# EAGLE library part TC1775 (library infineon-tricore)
TC1775 (AUDO1) 32-bit microcontroller for high demanding automotive and industrial applications (e.g. engine management, starter generator, 3-phase motor control or robotics) Source: http://www.infineon.com ..
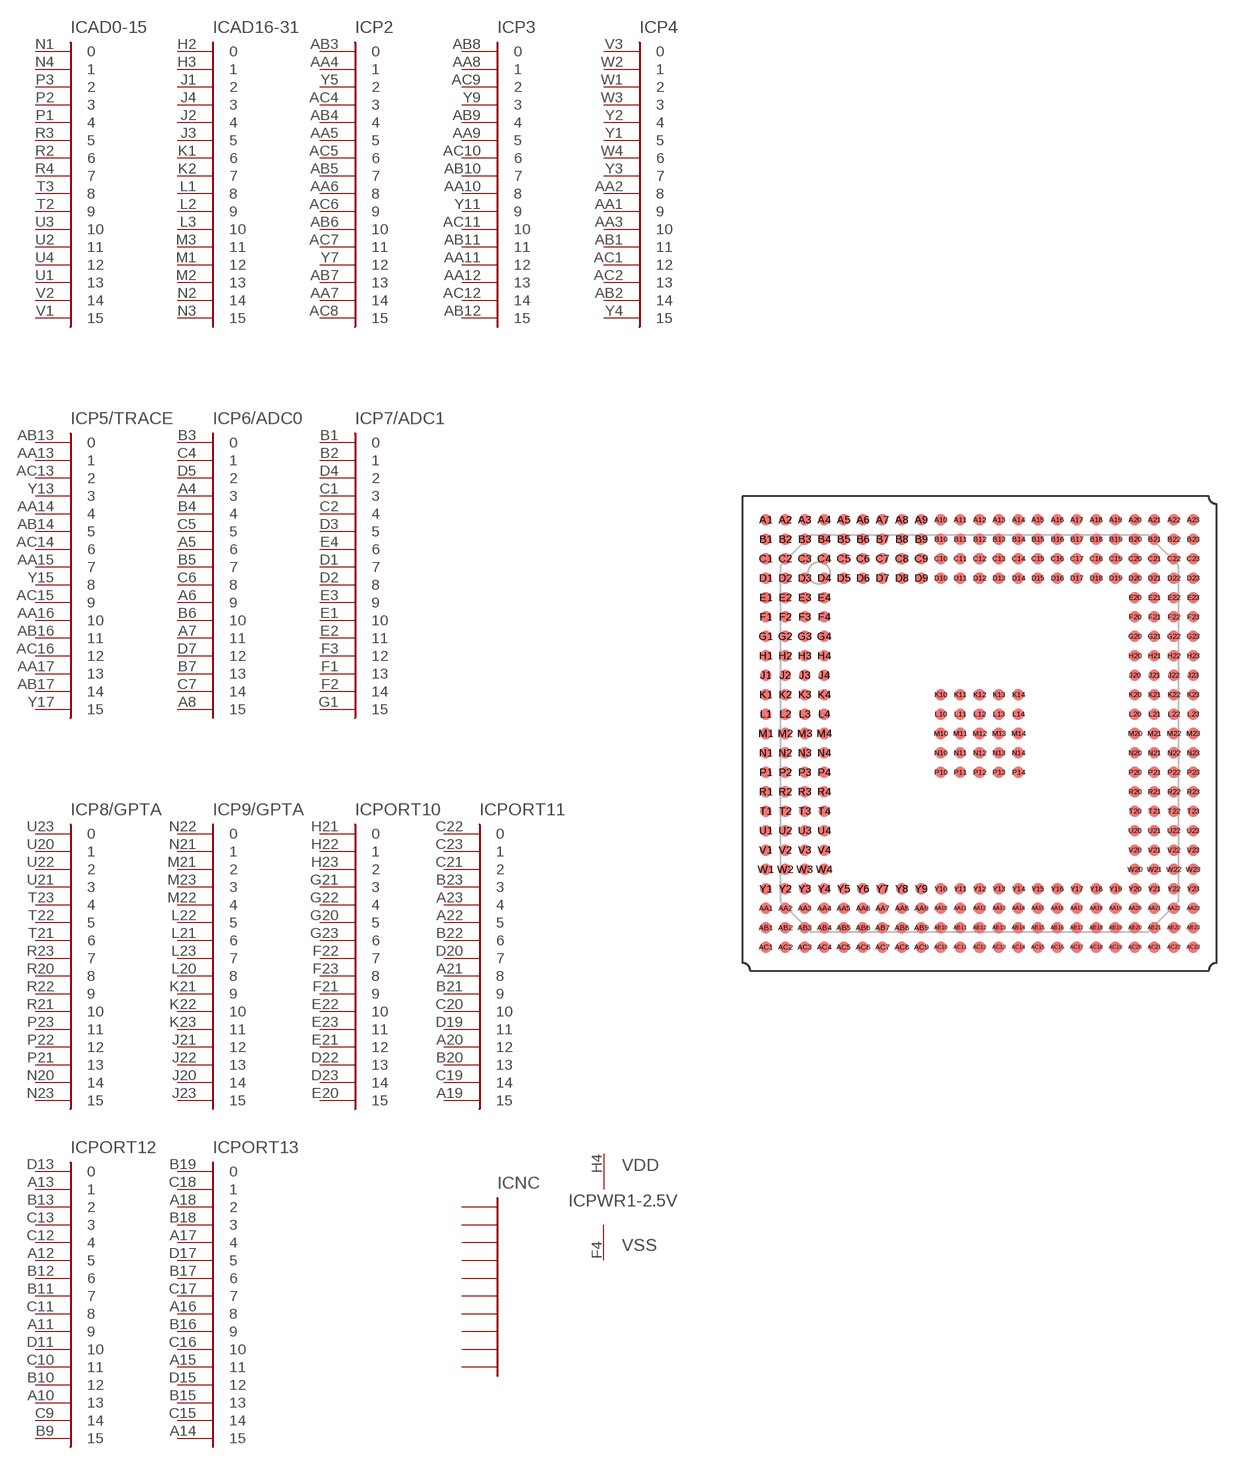
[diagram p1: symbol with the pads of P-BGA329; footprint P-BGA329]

Designator prefix IC; gates PORT12=PORT16 PORT13=PORT16 P8/GPTA=PORT16 P9/GPTA=PORT16 PORT10=PORT16 PORT11=PORT16 P5/TRACE=PORT16 P6/ADC0=PORT16 P7/ADC1=PORT16 AD0-15=PORT16 AD16-31=PORT16 P2=PORT16 P3=PORT16 P4=PORT16 NC=NC10 PWR1-2.5V=VSS_VDD PWR2-2.5V=VSS_VDD PWR3-2.5V=VSS_VDD PWR4-2.5V=VSS_VDD PWR5-2.5V=VSS_VDD PWR6-3.3V=VSS_VDD PWR7-3.3V=VSS_VDD PWR8-3.3V=VSS_VDD PWR9-3.3V=VSS_VDD PWR10-3.3V=VSS_VDD PWR11-3.3V=VSS_VDD PWR12-2.5V=VSS_VDD PWR13-2.5V=VSS_VDD PWR14-2.5V=VSS_VDD PWR15-2.5V=VSS_VDD P-SB-2.5V=VSS_VDD P-SRAM1-2.5V=VSS_VDD P-SRAM2-2.5V=VSS_VDD PWR16-2.5V=VSS_VDD PWR17-2.5V=VSS_VDD PWR18-2.5V=VSS_VDD PWR19-2.5V=VSS_VDD PWR20-2.5V=VSS_VDD PWR21-2.5V=VSS_VDD P-SC-5V=VSS_VDD P-DM-5V=VSS_VDD JTAG=JTAG-OCSD A=TC1775 PWR22=VSS PWR23=VSS PWR24=VSS PWR25=VSS PWR26=VSS

## TC1775 (OC_FARNELL: unknown; OC_NEWARK: unknown)  [P-BGA329]
A1  P-SC-5V:VDD  pwr
A2  P-SC-5V:VSS  pwr
A3  P-SRAM2-2.5V:VSS  pwr
A4  P6/ADC0:3  in
A5  P6/ADC0:6  in
A6  P6/ADC0:9  in
A7  P6/ADC0:11  in
A8  P6/ADC0:15  in
A9  A:VSSA  pwr
A10  PORT12:13  in
A11  PORT12:9  in
A12  PORT12:5  in
A13  PORT12:1  in
A14  PORT13:15  in
A15  PORT13:11  in
A16  PORT13:8  in
A17  PORT13:4  in
A18  PORT13:2  in
A19  PORT11:15  in
A20  PORT11:12  in
A21  PORT11:8  in
A22  PORT11:5  in
A23  PORT11:4  in
AA1  P4:9  in
AA2  P4:8  in
AA3  P4:10  in
AA4  P2:1  in
AA5  P2:5  in
AA6  P2:8  in
AA7  P2:14  in
AA8  P3:1  in
AA9  P3:5  in
AA10  P3:8  in
AA11  P3:12  in
AA12  P3:13  in
AA13  P5/TRACE:1  in
AA14  P5/TRACE:4  in
AA15  P5/TRACE:7  in
AA16  P5/TRACE:10  in
AA17  P5/TRACE:13  in
AA18  JTAG:TDO  out
AA19  JTAG:!TRST  in
AA20  A:XTAL4
AA21  A:VSS  pwr
AA22  A:VDD  pwr
AA23  A:VSS  pwr
AB1  P4:11  in
AB2  P4:14  in
AB3  P2:0  in
AB4  P2:4  in
AB5  P2:7  in
AB6  P2:10  in
AB7  P2:13  in
AB8  P3:0  in
AB9  P3:4  in
AB10  P3:7  in
AB11  P3:11  in
AB12  P3:15  in
AB13  P5/TRACE:0  in
AB14  P5/TRACE:5  in
AB15  NC:NC  nc
AB16  P5/TRACE:11  in
AB17  P5/TRACE:14  in
AB18  P-SRAM2-2.5V:VDD  pwr
AB19  JTAG:TCK  in
AB20  JTAG:TMS  in
AB21  A:XTAL3
AB22  NC:NC  nc
AB23  A:TESTMODE
AC1  P4:12  in
AC2  P4:13  in
AC3  NC:NC  nc
AC4  P2:3  in
AC5  P2:6  in
AC6  P2:9  in
AC7  P2:11  in
AC8  P2:15  in
AC9  P3:2  in
AC10  P3:6  in
AC11  P3:10  in
AC12  P3:14  in
AC13  P5/TRACE:2  in
AC14  P5/TRACE:6  in
AC15  P5/TRACE:9  in
AC16  P5/TRACE:12  in
AC17  P-SRAM1-2.5V:VDD  pwr
AC18  JTAG:!BRKOUT  out
AC19  JTAG:TDI  in
AC20  JTAG:!BRKIN  in
AC21  A:VDD  pwr
AC22  A:XTAL2
AC23  A:XTAL1
B1  P7/ADC1:0  in
B2  P7/ADC1:1  in
B3  P6/ADC0:0  in
B4  P6/ADC0:4  in
B5  P6/ADC0:7  in
B6  P6/ADC0:10  in
B7  P6/ADC0:13  in
B8  A:VAGND  pwr
B9  PORT12:15  in
B10  PORT12:12  in
B11  PORT12:7  in
B12  PORT12:6  in
B13  PORT12:2  in
B14  P-SB-2.5V:VDD  pwr
B15  PORT13:13  in
B16  PORT13:9  in
B17  PORT13:6  in
B18  PORT13:3  in
B19  PORT13:0  in
B20  PORT11:13  in
B21  PORT11:9  in
B22  PORT11:6  in
B23  PORT11:3  in
C1  P7/ADC1:3  in
C2  P7/ADC1:4  in
C3  P-DM-5V:VDD  pwr
C4  P6/ADC0:1  in
C5  P6/ADC0:5  in
C6  P6/ADC0:8  in
C7  P6/ADC0:14  in
C8  A:VAREF  pwr
C9  PORT12:14  in
C10  PORT12:11  in
C11  PORT12:8  in
C12  PORT12:4  in
C13  PORT12:3  in
C14  NC:NC  nc
C15  PORT13:14  in
C16  PORT13:10  in
C17  PORT13:7  in
C18  PORT13:1  in
C19  PORT11:14  in
C20  PORT11:10  in
C21  PORT11:2  in
C22  PORT11:0  in
C23  PORT11:1  in
D1  P7/ADC1:7  in
D2  P7/ADC1:8  in
D3  P7/ADC1:5  in
D4  P7/ADC1:2  in
D5  P6/ADC0:2  in
D6  PWR15-2.5V:VDD  pwr
D7  P6/ADC0:12  in
D8  PWR6-3.3V:VDD  pwr
D9  A:VDDA  pwr
D10  NC:NC  nc
D11  PORT12:10  in
D12  PWR7-3.3V:VDD  pwr
D13  PORT12:0  in
D14  PWR16-2.5V:VDD  pwr
D15  PORT13:12  in
D16  PWR8-3.3V:VDD  pwr
D17  PORT13:5  in
D18  PWR4-2.5V:VSS  pwr
D19  PORT11:11  in
D20  PORT11:7  in
D21  NC:NC  nc
D22  PORT10:13  in
D23  PORT10:14  in
E1  P7/ADC1:10  in
E2  P7/ADC1:11  in
E3  P7/ADC1:9  in
E4  P7/ADC1:6  in
E20  PORT10:15  in
E21  PORT10:12  in
E22  PORT10:10  in
E23  PORT10:11  in
F1  P7/ADC1:13  in
F2  P7/ADC1:14  in
F3  P7/ADC1:12  in
F4  PWR1-2.5V:VSS  pwr
F20  PWR19-2.5V:VDD  pwr
F21  PORT10:9  in
F22  PORT10:7  in
F23  PORT10:8  in
G1  P7/ADC1:15  in
G2  A:VAREF  pwr
G3  A:VSSA  pwr
G4  A:VAGND  pwr
G20  PORT10:5  in
G21  PORT10:3  in
G22  PORT10:4  in
G23  PORT10:6  in
H1  A:VDDA  pwr
H2  AD16-31:0  in
H3  AD16-31:1  in
H4  PWR1-2.5V:VDD  pwr
H20  PWR9-3.3V:VDD  pwr
H21  PORT10:0  in
H22  PORT10:1  in
H23  PORT10:2  in
J1  AD16-31:2  in
J2  AD16-31:4  in
J3  AD16-31:5  in
J4  AD16-31:3  in
J20  P9/GPTA:14  in
J21  P9/GPTA:12  in
J22  P9/GPTA:13  in
J23  P9/GPTA:15  in
K1  AD16-31:6  in
K2  AD16-31:7  in
K3  NC:NC  nc
K4  PWR12-2.5V:VDD  pwr
K10  PWR5-2.5V:VSS  pwr
K11  PWR6-3.3V:VSS  pwr
K12  PWR7-3.3V:VSS  pwr
K13  PWR8-3.3V:VSS  pwr
K14  PWR9-3.3V:VSS  pwr
K20  PWR20-2.5V:VDD  pwr
K21  P9/GPTA:9  in
K22  P9/GPTA:10  in
K23  P9/GPTA:11  in
L1  AD16-31:8  in
L2  AD16-31:9  in
L3  AD16-31:10  in
L4  NC:NC  nc
L10  PWR10-3.3V:VSS  pwr
L11  PWR11-3.3V:VSS  pwr
L12  PWR12-2.5V:VSS  pwr
L13  PWR13-2.5V:VSS  pwr
L14  PWR14-2.5V:VSS  pwr
L20  P9/GPTA:8  in
L21  P9/GPTA:6  in
L22  P9/GPTA:5  in
L23  P9/GPTA:7  in
M1  AD16-31:12  in
M2  AD16-31:13  in
M3  AD16-31:11  in
M4  PWR2-2.5V:VDD  pwr
M10  PWR16-2.5V:VSS  pwr
M11  PWR17-2.5V:VSS  pwr
M12  PWR18-2.5V:VSS  pwr
M13  PWR19-2.5V:VSS  pwr
M14  PWR20-2.5V:VSS  pwr
M20  PWR10-3.3V:VDD  pwr
M21  P9/GPTA:2  in
M22  P9/GPTA:4  in
M23  P9/GPTA:3  in
N1  AD0-15:0  in
N2  AD16-31:14  in
N3  AD16-31:15  in
N4  AD0-15:1  in
N10  PWR25:VSS  pwr
N11  PWR26:VSS  pwr
N12  P-DM-5V:VSS  pwr
N13  P-SB-2.5V:VSS  pwr
N14  P-SRAM1-2.5V:VSS  pwr
N20  P8/GPTA:14  in
N21  P9/GPTA:1  in
N22  P9/GPTA:0  in
N23  P8/GPTA:15  in
P1  AD0-15:4  in
P2  AD0-15:3  in
P3  AD0-15:2  in
P4  PWR13-2.5V:VDD  pwr
P10  PWR15-2.5V:VSS  pwr
P11  PWR22:VSS  pwr
P12  PWR23:VSS  pwr
P13  PWR21-2.5V:VSS  pwr
P14  PWR24:VSS  pwr
P20  PWR21-2.5V:VDD  pwr
P21  P8/GPTA:13  in
P22  P8/GPTA:12  in
P23  P8/GPTA:11  in
R1  A:CLKOUT  out
R2  AD0-15:6  in
R3  AD0-15:5  in
R4  AD0-15:7  in
R20  P8/GPTA:8  in
R21  P8/GPTA:10  in
R22  P8/GPTA:9  in
R23  P8/GPTA:7  in
T1  A:CLKIN  in
T2  AD0-15:9  in
T3  AD0-15:8  in
T4  PWR3-2.5V:VDD  pwr
T20  PWR11-3.3V:VDD  pwr
T21  P8/GPTA:6  in
T22  P8/GPTA:5  in
T23  P8/GPTA:4  in
U1  AD0-15:13  in
U2  AD0-15:11  in
U3  AD0-15:10  in
U4  AD0-15:12  in
U20  P8/GPTA:1  in
U21  P8/GPTA:3  in
U22  P8/GPTA:2  in
U23  P8/GPTA:0  in
V1  AD0-15:15  in
V2  AD0-15:14  in
V3  P4:0  in
V4  PWR14-2.5V:VDD  pwr
V20  PWR3-2.5V:VSS  pwr
V21  A:CLKSEL0  in
V22  A:CLKSEL2  in
V23  A:CLKSEL1  in
W1  P4:2  in
W2  P4:1  in
W3  P4:3  in
W4  P4:6  in
W20  A:HDRST
W21  A:CFG2  in
W22  A:BYPASS  in
W23  A:CFG3  in
Y1  P4:5  in
Y2  P4:4  in
Y3  P4:7  in
Y4  P4:15  in
Y5  P2:2  in
Y6  PWR2-2.5V:VSS  pwr
Y7  P2:12  in
Y8  PWR4-2.5V:VDD  pwr
Y9  P3:3  in
Y10  PWR17-2.5V:VDD  pwr
Y11  P3:9  in
Y12  PWR5-2.5V:VDD  pwr
Y13  P5/TRACE:3  in
Y14  NC:NC  nc
Y15  P5/TRACE:8  in
Y16  NC:NC  nc
Y17  P5/TRACE:15  in
Y18  PWR18-2.5V:VDD  pwr
Y19  JTAG:!OCDSE  in
Y20  A:NMI  in
Y21  A:PORST  in
Y22  A:CFG1  in
Y23  A:CFG0  in

## Footprint P-BGA329 (pad centres in mm)
P-BGA-329 Plastic Ball Grid Array Package Source: http://www.infineon.com
smd 0.76 x 0.76: A1 -13.97,13.97; A2 -12.7,13.97; A3 -11.43,13.97; A4 -10.16,13.97; A5 -8.89,13.97; A6 -7.62,13.97; A7 -6.35,13.97; A8 -5.08,13.97; A9 -3.81,13.97; A10 -2.54,13.97; A11 -1.27,13.97; A12 0,13.97; A13 1.27,13.97; A14 2.54,13.97; A15 3.81,13.97; A16 5.08,13.97; A17 6.35,13.97; A18 7.62,13.97; A19 8.89,13.97; A20 10.16,13.97; A21 11.43,13.97; A22 12.7,13.97; A23 13.97,13.97; AA1 -13.97,-11.43; AA2 -12.7,-11.43; AA3 -11.43,-11.43; AA4 -10.16,-11.43; AA5 -8.89,-11.43; AA6 -7.62,-11.43; AA7 -6.35,-11.43; AA8 -5.08,-11.43; AA9 -3.81,-11.43; AA10 -2.54,-11.43; AA11 -1.27,-11.43; AA12 0,-11.43; AA13 1.27,-11.43; AA14 2.54,-11.43; AA15 3.81,-11.43; AA16 5.08,-11.43; AA17 6.35,-11.43; AA18 7.62,-11.43; AA19 8.89,-11.43; AA20 10.16,-11.43; AA21 11.43,-11.43; AA22 12.7,-11.43; AA23 13.97,-11.43; AB1 -13.97,-12.7; AB2 -12.7,-12.7; AB3 -11.43,-12.7; AB4 -10.16,-12.7; AB5 -8.89,-12.7; AB6 -7.62,-12.7; AB7 -6.35,-12.7; AB8 -5.08,-12.7; AB9 -3.81,-12.7; AB10 -2.54,-12.7; AB11 -1.27,-12.7; AB12 0,-12.7; AB13 1.27,-12.7; AB14 2.54,-12.7; AB15 3.81,-12.7; AB16 5.08,-12.7; AB17 6.35,-12.7; AB18 7.62,-12.7; AB19 8.89,-12.7; AB20 10.16,-12.7; AB21 11.43,-12.7; AB22 12.7,-12.7; AB23 13.97,-12.7; AC1 -13.97,-13.97; AC2 -12.7,-13.97; AC3 -11.43,-13.97; AC4 -10.16,-13.97; AC5 -8.89,-13.97; AC6 -7.62,-13.97; AC7 -6.35,-13.97; AC8 -5.08,-13.97; AC9 -3.81,-13.97; AC10 -2.54,-13.97; AC11 -1.27,-13.97; AC12 0,-13.97; AC13 1.27,-13.97; AC14 2.54,-13.97; AC15 3.81,-13.97; AC16 5.08,-13.97; AC17 6.35,-13.97; AC18 7.62,-13.97; AC19 8.89,-13.97; AC20 10.16,-13.97; AC21 11.43,-13.97; AC22 12.7,-13.97; AC23 13.97,-13.97; B1 -13.97,12.7; B2 -12.7,12.7; B3 -11.43,12.7; B4 -10.16,12.7; B5 -8.89,12.7; B6 -7.62,12.7; B7 -6.35,12.7; B8 -5.08,12.7; B9 -3.81,12.7; B10 -2.54,12.7; B11 -1.27,12.7; B12 0,12.7; B13 1.27,12.7; B14 2.54,12.7; B15 3.81,12.7; B16 5.08,12.7; B17 6.35,12.7; B18 7.62,12.7; B19 8.89,12.7; B20 10.16,12.7; B21 11.43,12.7; B22 12.7,12.7; B23 13.97,12.7; C1 -13.97,11.43; C2 -12.7,11.43; C3 -11.43,11.43; C4 -10.16,11.43; C5 -8.89,11.43; C6 -7.62,11.43; C7 -6.35,11.43; C8 -5.08,11.43; C9 -3.81,11.43; C10 -2.54,11.43; C11 -1.27,11.43; C12 0,11.43; C13 1.27,11.43; C14 2.54,11.43; C15 3.81,11.43; C16 5.08,11.43; C17 6.35,11.43; C18 7.62,11.43; C19 8.89,11.43; C20 10.16,11.43; C21 11.43,11.43; C22 12.7,11.43; C23 13.97,11.43; D1 -13.97,10.16; D2 -12.7,10.16; D3 -11.43,10.16; D4 -10.16,10.16; D5 -8.89,10.16; D6 -7.62,10.16; D7 -6.35,10.16; D8 -5.08,10.16; D9 -3.81,10.16; D10 -2.54,10.16; D11 -1.27,10.16; D12 0,10.16; D13 1.27,10.16; D14 2.54,10.16; D15 3.81,10.16; D16 5.08,10.16; D17 6.35,10.16; D18 7.62,10.16; D19 8.89,10.16; D20 10.16,10.16; D21 11.43,10.16; D22 12.7,10.16; D23 13.97,10.16; E1 -13.97,8.89; E2 -12.7,8.89; E3 -11.43,8.89; E4 -10.16,8.89; E20 10.16,8.89; E21 11.43,8.89; E22 12.7,8.89; E23 13.97,8.89; F1 -13.97,7.62; F2 -12.7,7.62; F3 -11.43,7.62; F4 -10.16,7.62; F20 10.16,7.62; F21 11.43,7.62; F22 12.7,7.62; F23 13.97,7.62; G1 -13.97,6.35; G2 -12.7,6.35; G3 -11.43,6.35; G4 -10.16,6.35; G20 10.16,6.35; G21 11.43,6.35; G22 12.7,6.35; G23 13.97,6.35; H1 -13.97,5.08; H2 -12.7,5.08; H3 -11.43,5.08; H4 -10.16,5.08; H20 10.16,5.08; H21 11.43,5.08; H22 12.7,5.08; H23 13.97,5.08; J1 -13.97,3.81; J2 -12.7,3.81; J3 -11.43,3.81; J4 -10.16,3.81; J20 10.16,3.81; J21 11.43,3.81; J22 12.7,3.81; J23 13.97,3.81; K1 -13.97,2.54; K2 -12.7,2.54; K3 -11.43,2.54; K4 -10.16,2.54; K10 -2.54,2.54; K11 -1.27,2.54; K12 0,2.54; K13 1.27,2.54; K14 2.54,2.54; K20 10.16,2.54; K21 11.43,2.54; K22 12.7,2.54; K23 13.97,2.54; L1 -13.97,1.27; L2 -12.7,1.27; L3 -11.43,1.27; L4 -10.16,1.27; L10 -2.54,1.27; L11 -1.27,1.27; L12 0,1.27; L13 1.27,1.27; L14 2.54,1.27; L20 10.16,1.27; L21 11.43,1.27; L22 12.7,1.27; L23 13.97,1.27; M1 -13.97,0; M2 -12.7,0; M3 -11.43,0; M4 -10.16,0; M10 -2.54,0; M11 -1.27,0; M12 0,0; M13 1.27,0; M14 2.54,0; M20 10.16,0; M21 11.43,0; M22 12.7,0; M23 13.97,0; N1 -13.97,-1.27; N2 -12.7,-1.27; N3 -11.43,-1.27; N4 -10.16,-1.27; N10 -2.54,-1.27; N11 -1.27,-1.27; N12 0,-1.27; N13 1.27,-1.27; N14 2.54,-1.27; N20 10.16,-1.27; N21 11.43,-1.27; N22 12.7,-1.27; N23 13.97,-1.27; P1 -13.97,-2.54; P2 -12.7,-2.54; P3 -11.43,-2.54; P4 -10.16,-2.54; P10 -2.54,-2.54; P11 -1.27,-2.54; P12 0,-2.54; P13 1.27,-2.54; P14 2.54,-2.54; P20 10.16,-2.54; P21 11.43,-2.54; P22 12.7,-2.54; P23 13.97,-2.54; R1 -13.97,-3.81; R2 -12.7,-3.81; R3 -11.43,-3.81; R4 -10.16,-3.81; R20 10.16,-3.81; R21 11.43,-3.81; R22 12.7,-3.81; R23 13.97,-3.81; T1 -13.97,-5.08; T2 -12.7,-5.08; T3 -11.43,-5.08; T4 -10.16,-5.08; T20 10.16,-5.08; T21 11.43,-5.08; T22 12.7,-5.08; T23 13.97,-5.08; U1 -13.97,-6.35; U2 -12.7,-6.35; U3 -11.43,-6.35; U4 -10.16,-6.35; U20 10.16,-6.35; U21 11.43,-6.35; U22 12.7,-6.35; U23 13.97,-6.35; V1 -13.97,-7.62; V2 -12.7,-7.62; V3 -11.43,-7.62; V4 -10.16,-7.62; V20 10.16,-7.62; V21 11.43,-7.62; V22 12.7,-7.62; V23 13.97,-7.62; W1 -13.97,-8.89; W2 -12.7,-8.89; W3 -11.43,-8.89; W4 -10.16,-8.89; W20 10.16,-8.89; W21 11.43,-8.89; W22 12.7,-8.89; W23 13.97,-8.89; Y1 -13.97,-10.16; Y2 -12.7,-10.16; Y3 -11.43,-10.16; Y4 -10.16,-10.16; Y5 -8.89,-10.16; Y6 -7.62,-10.16; Y7 -6.35,-10.16; Y8 -5.08,-10.16; Y9 -3.81,-10.16; Y10 -2.54,-10.16; Y11 -1.27,-10.16; Y12 0,-10.16; Y13 1.27,-10.16; Y14 2.54,-10.16; Y15 3.81,-10.16; Y16 5.08,-10.16; Y17 6.35,-10.16; Y18 7.62,-10.16; Y19 8.89,-10.16; Y20 10.16,-10.16; Y21 11.43,-10.16; Y22 12.7,-10.16; Y23 13.97,-10.16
